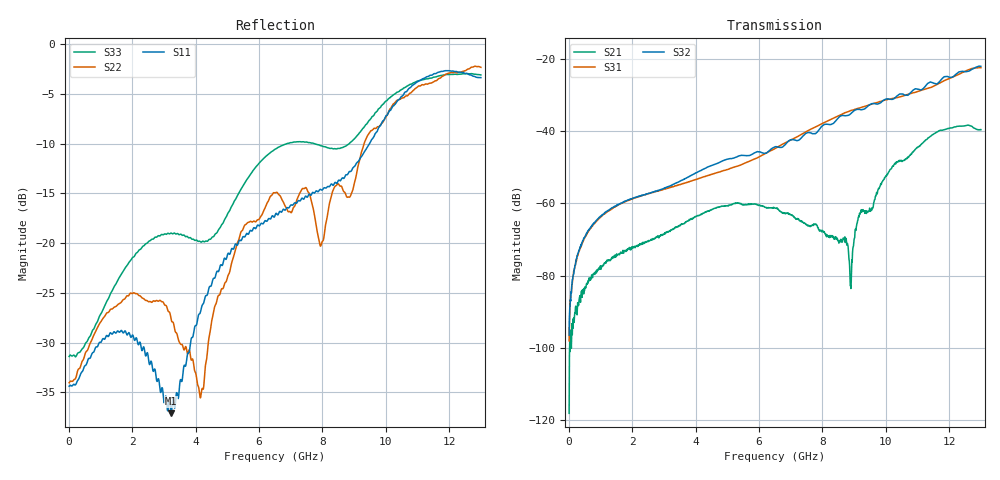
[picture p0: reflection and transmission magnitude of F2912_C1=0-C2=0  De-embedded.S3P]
! Integrated Device Technology
! Corporate Headquarters
! 6024 Silver Creek Valley Road
! San Jose, CA 95138  USA
! Phone:  1-408-284-8200
! Toll Free:  1-800-223-1366
! Webpage:  http://www.idt.com/
! Timing and RF Division
! 515 Groton Road, Suite 102
! Westford, MA 01886-6024
! Device:  F2912
! Description: High Reliability SP2T RF Switch
! Frequency:  9 kHz -  9 GHz
! Package:  4x4 mm QFN Plastic Package: 20 pin
! Ports:  3 RF, 5 DC
!  Pin  1  = GND
!  Pin  2  = GND
!  Pin  3  = RF1  =  Port 1
!  Pin  4  = GND
!  Pin  5  = GND
!  Pin  6  = GND
!  Pin  7  = GND
!  Pin  8  = RF_COM =  Port 3
!  Pin  9  = GND
!  Pin 10  = GND
!  Pin 11  = GND
!  Pin 12  = GND
!  Pin 13  = RF2  =  Port 2
!  Pin 14  = GND
!  Pin 15  = GND
!  Pin 16  = CTL2
!  Pin 17  = CTL1
!  Pin 18  = LogicCTL
!  Pin 19  = ModeCTL
!  Pin 20  = Vcc
! Logic:  3.3 V
! Mode:  2 pin control
! Voltage:  +3.30  Volts
! Current:  0.034 mA
! State:  All Off
! CTL1:  Logic LOW
! CTL2:  Logic LOW
! Data:  The device was measured on a F2912 evaluation board which has
!  individual transmission lines to the RF pins.  Data was collected
!  using a calibrated network analyzer.  The evaluation board was
!  de-embedded using AFR (Keysight).
!  The reference plane is the edge of the package pin.
! Misc:  Action Tracker AT0438
! Date Measured:  2018-12-14
! Date:  2018-12-14  MJV
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# Hz S dB R 50
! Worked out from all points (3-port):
!   1300 points, 10 MHz to 13 GHz, reference 50 ohm
!   strongest paths, dB at 10 MHz, 3.26 GHz, 6.51 GHz, 9.76 GHz, 13 GHz:
!     S32: -96.5, -54.9, -44.4, -32.5, -22.1
!     S31: -98.0, -55.5, -44.8, -32.0, -22.5
!     S21: -118.0, -67.2, -61.4, -56.2, -39.6
!   lowest |S11| = -37.1 dB at 3.23 GHz (marker M1), VSWR 1.03, Z = 48.6 + j0.0777 ohm
!   |S11| at or under -10 dB: start of sweep to 9.486 GHz
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1e7  -34.38 179.0  -98.15 153.2  -99.66 114.6
     -118.04 -142.8  -34.03 178.8  -90.40 49.7
     -98.01 74.0  -96.46 57.3  -31.40 179.9
9.9e8  -29.96 158.3  -77.74 90.0  -63.89 89.5
       -77.52 90.5  -27.99 150.0  -63.57 89.8
       -63.94 89.7  -63.70 89.5  -27.22 -166.1
3.23e9  -37.11 176.7  -67.25 105.8  -55.56 106.3
        -67.42 105.8  -27.66 -138.0  -55.01 114.6
        -55.54 106.0  -55.04 114.6  -18.98 -126.8
4.19e9  -26.41 140.5  -62.85 102.0  -52.88 118.9
        -62.98 102.3  -34.81 168.9  -50.83 126.4
        -52.85 119.4  -50.80 126.2  -19.88 -139.8
6.51e9  -17.17 173.5  -61.11 90.9  -44.85 158.2
        -61.36 91.1  -14.95 -177.0  -44.72 142.5
        -44.81 158.1  -44.36 143.2  -10.54 -170.3
8.7e9  -13.38 159.7  -69.23 -146.1  -35.05 152.9
       -69.74 -157.8  -14.87 166.6  -35.75 150.8
       -35.03 152.8  -35.78 152.1  -10.29 170.2
8.89e9  -12.79 155.8  -86.65 -120.4  -34.39 148.8
        -82.73 -94.2  -15.22 153.4  -35.18 148.8
        -34.38 148.9  -35.26 146.8  -9.85 163.2
9.2e9  -11.43 147.6  -62.71 -61.3  -33.57 143.2
       -62.62 -57.7  -11.28 140.0  -34.05 145.2
       -33.57 143.2  -34.10 147.6  -8.80 153.5
1.022e10  -6.23 135.4  -49.64 -29.0  -30.98 123.7
          -49.76 -29.9  -6.08 146.0  -30.86 128.9
          -30.97 123.7  -31.22 128.3  -5.13 142.9
1.3e10  -3.35 118.3  -38.97 172.6  -22.50 73.6
        -39.63 179.5  -2.32 127.5  -22.84 79.4
        -22.53 73.4  -22.14 81.2  -3.09 137.6
